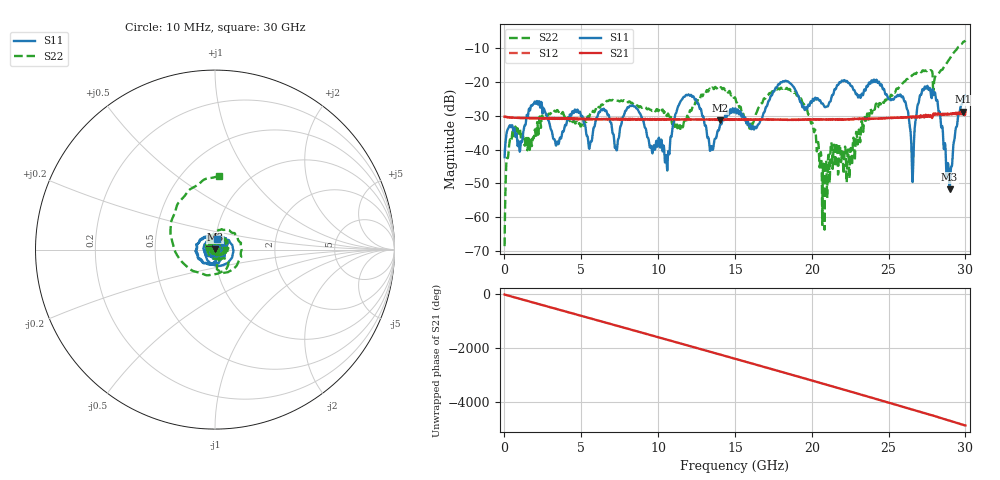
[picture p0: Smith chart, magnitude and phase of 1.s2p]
! 5/14/2024 1:27:12 PM
! D:\_XLC\DA9-3050-0-26.5G-2812\1.S2P
! CHANNEL.1
! TR.MEASUREMENT
! CORRECTED.DATA
! RF.CORRECTION: FULL.TWO.PORT.CAL.PORT.1.2
! AVERAGING.OFF
! IF.BANDWIDTH: 1KHZ
! SWEEPTYPE:  FREQ.SWEEP(Linear)
! Reference Plane Port Info
! PORT:  PORT1  PORT2
! DISTANCE:  0  m  0  m
! TIME:  0  s  0  s
! PHASE.OFFSET:  0 °  0 °
! LOSS:  0  dB  0  dB
! REF.LOSS:  0  dB  0  dB
! REF.FREQ:  0  Hz  0  Hz
! Power Info
! POWER:  -10  dBm  -10  dBm
! EFF.POWER:  -10  dBm  -10  dBm
! SOURCE.ATTEN:  0  dB  0  dB
! TEST.ATTEN:  0  dB  0  dB
# GHZ S RI R 50.0
! FREQ.GHZ  S11RE  S11IM  S21RE  S21IM  S12RE  S12IM  S22RE  S22IM
!; PortSelection: Port_12
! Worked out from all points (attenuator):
!   1372 points, 10 MHz to 30 GHz, reference 50 ohm
!   highest |S21| = -28.72 dB at 29.87 GHz (marker M1); lowest = -31.3 dB at 14.03 GHz (marker M2)
!   lowest |S11| = -51.7 dB at 28.97 GHz (marker M3), VSWR 1.01, Z = 50 + j0.255 ohm
!   |S11| at or under -10 dB: start of sweep to end of sweep
!   |S22| runs from -68.5 to -7.7 dB; largest |S21 - S12| = 0.0035
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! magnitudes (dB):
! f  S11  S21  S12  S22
! 10 MHz  -42.2  -30.2  -30.2  -68.5
! 228.7 MHz  -33.9  -30.4  -30.4  -42.3
! 622.4 MHz  -33.7  -30.5  -30.5  -36.1
! 5.019 GHz  -30.2  -30.8  -30.9  -32.4
! 7.271 GHz  -39.6  -30.8  -31.0  -25.4
! 8.409 GHz  -27.2  -31.0  -31.0  -26.7
! 10.01 GHz  -37.6  -31.0  -31.0  -28.6
! 10.57 GHz  -45.2  -30.9  -31.1  -30.0
! 11.89 GHz  -23.9  -31.0  -31.0  -30.0
! 13.46 GHz  -38.9  -31.1  -31.1  -22.2
! 14.03 GHz  -32.6  -31.3  -31.1  -21.8
! 15.01 GHz  -27.8  -31.1  -31.1  -24.6
! 20 GHz  -26.1  -31.1  -31.0  -32.1
! 20.77 GHz  -26.8  -31.0  -31.1  -44.1
! 25.01 GHz  -24.8  -30.6  -30.6  -24.9
! 26.02 GHz  -25.7  -30.5  -30.5  -19.9
! 26.54 GHz  -48.7  -30.3  -30.3  -17.9
! 27.11 GHz  -23.8  -30.0  -30.1  -17.1
! 27.96 GHz  -23.5  -29.5  -29.3  -19.8
! 28.97 GHz  -51.7  -29.5  -29.4  -13.1
! 29.87 GHz  -25.0  -28.7  -29.6  -8.1
! 30 GHz  -24.1  -29.0  -29.6  -7.7
